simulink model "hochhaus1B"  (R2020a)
settings: Solver=ode45  StartTime=0.0  StopTime=2  MaxStep=1e-3  RelTol=1e-3  EnableMultiTasking=on

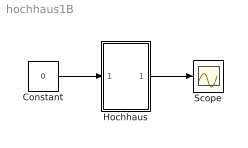
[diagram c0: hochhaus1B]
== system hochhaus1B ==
  Constant : Constant  Value=0
  Hochhaus : Subsystem  mask(Schwingerkette){m=[6,6,1]*1e3, c=[3,3,1]*1e6, x0=[0;0;0], v0=[0;0;10]}
      mask prompts: m "Massen"; c "Steifigkeiten"; x0 "Anfangsauslenkungen"; v0 "Anfangsgeschwindigkeiten"
      mask help: eindimensionale Schwingerkette mit oberem freien Ende und Krafterregung am Fusspunkt
  Scope : Scope
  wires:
  Hochhaus/1(x) -> Scope/1
  Constant/1 -> Hochhaus/1(F)

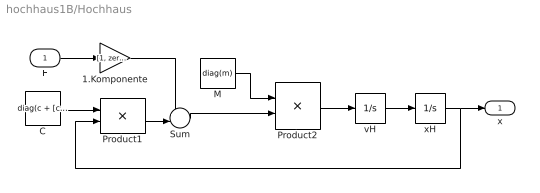
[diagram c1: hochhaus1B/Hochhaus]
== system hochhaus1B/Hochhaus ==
  F : Inport
  1.Komponente : Gain  Gain=[1, zeros(1,length(m)-1)]  SaturateOnIntegerOverflow=on
  C : Constant  Value=diag(c + [c(2:end),0]) - diag(c(2:end),1) - diag(c(2:end),-1)  VectorParams1D=off
  M : Constant  Value=diag(m)  VectorParams1D=off
  Product1 : Product  Multiplication=Matrix(*)  InputSameDT=on  SaturateOnIntegerOverflow=on
  Product2 : Product  Inputs=/*  Multiplication=Matrix(*)  InputSameDT=on  SaturateOnIntegerOverflow=on
  Sum : Sum  Inputs=+-|  InputSameDT=on  SaturateOnIntegerOverflow=on
  vH : Integrator  InitialCondition=v0
  xH : Integrator  InitialCondition=x0
  x : Outport
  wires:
  1.Komponente/1 -> Sum/1
  F/1 -> 1.Komponente/1
  M/1 -> Product2/1
  Product2/1 -> vH/1
  Sum/1 -> Product2/2
  C/1 -> Product1/1
  Product1/1 -> Sum/2
  xH/1 -> x/1, Product1/2
  vH/1 -> xH/1
